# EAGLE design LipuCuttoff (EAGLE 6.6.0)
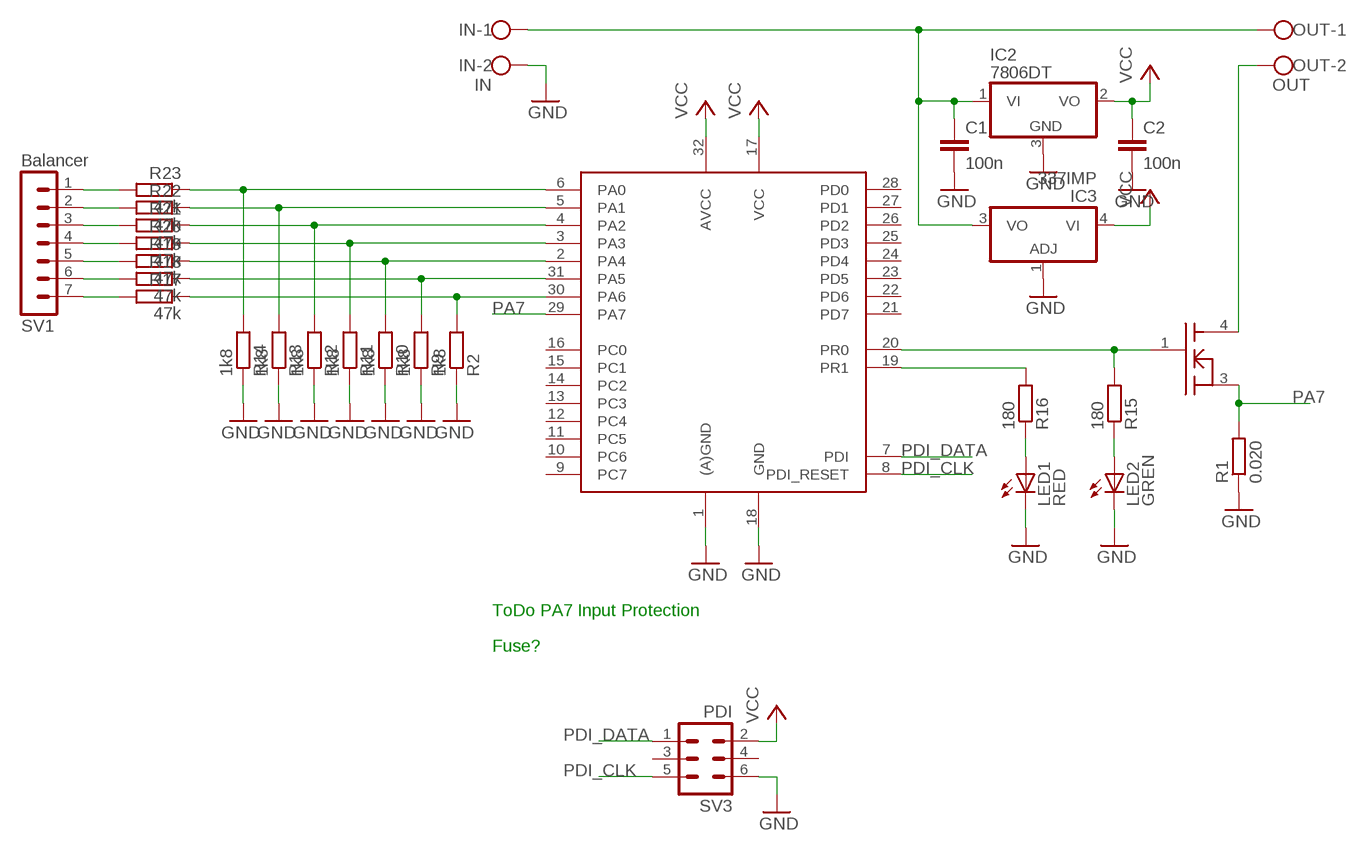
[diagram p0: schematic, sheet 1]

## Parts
C1  100n  C-EUC0805  [C0805]
C2  100n  C-EUC0805  [C0805]
IC2  7806DT  [TO252]
IC3  337IMP  [SOT223]
IN  IN  W237-102  [W237-102]
LED1  RED  LEDSML0805  [SML0805]
LED2  GREN  LEDSML0805  [SML0805]
OUT  OUT  W237-102  [W237-102]
R1  0.020  R-EU_R2512  [R2512]
R2  1k8  R-EU_M0805  [M0805]
R9  1k8  R-EU_M0805  [M0805]
R10  1k8  R-EU_M0805  [M0805]
R11  1k8  R-EU_M0805  [M0805]
R12  1k8  R-EU_M0805  [M0805]
R13  1k8  R-EU_M0805  [M0805]
R14  1k8  R-EU_M0805  [M0805]
R15  180  R-EU_M0805  [M0805]
R16  180  R-EU_M0805  [M0805]
R17  47k  R-EU_M0805  [M0805]
R18  47k  R-EU_M0805  [M0805]
R19  47k  R-EU_M0805  [M0805]
R20  47k  R-EU_M0805  [M0805]
R21  47k  R-EU_M0805  [M0805]
R22  47k  R-EU_M0805  [M0805]
R23  47k  R-EU_M0805  [M0805]
SV1  Balancer  MA07-1  [MA07-1]
SV3  PDI  MA03-2  [MA03-2]
U$1  ATXMEGA8E5  [TQFP-32]
U$2  95N2LH5  [DPAK]

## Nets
GND: C1.2 C2.2 IC2.3(GND) IC3.1(ADJ) IN.2 LED1.C LED2.C R1.1 R2.1 R9.1 R10.1 R11.1 R12.1 R13.1 R14.1 SV3.6 U$1.1((A)GND) U$1.18(GND)
N$1: R17.2 SV1.7
N$2: R18.2 SV1.6
N$3: R9.2 R18.1 U$1.31(PA5)
N$4: R19.2 SV1.5
N$5: R11.2 R20.1 U$1.3(PA3)
N$6: R20.2 SV1.4
N$7: R13.2 R22.1 U$1.5(PA1)
N$8: R21.2 SV1.3
N$9: R22.2 SV1.2
N$10: R23.2 SV1.1
N$12: OUT.2 U$2.4(D)
N$13: C1.1 IC2.1(VI) IC3.3(VO) IN.1 OUT.1
N$15: LED2.A R15.1
N$16: R16.2 U$1.19(PR1)
N$17: LED1.A R16.1
N$18: R15.2 U$1.20(PR0) U$2.1(G)
N$19: R2.2 R17.1 U$1.30(PA6)
N$21: R10.2 R19.1 U$1.2(PA4)
N$23: R12.2 R21.1 U$1.4(PA2)
N$25: R14.2 R23.1 U$1.6(PA0)
PA7: R1.2 U$1.29(PA7) U$2.3(S)
PDI_CLK: SV3.5 U$1.8(PDI_RESET)
PDI_DATA: SV3.1 U$1.7(PDI)
VCC: C2.1 IC2.2(VO) IC3.4(VI) SV3.2 U$1.17(VCC) U$1.32(AVCC)
Unconnected: SV3.3 SV3.4 U$1.9(PC7) U$1.10(PC6) U$1.11(PC5) U$1.12(PC4) U$1.13(PC3) U$1.14(PC2) U$1.15(PC1) U$1.16(PC0) U$1.21(PD7) U$1.22(PD6) U$1.23(PD5) U$1.24(PD4) U$1.25(PD3) U$1.26(PD2) U$1.27(PD1) U$1.28(PD0)

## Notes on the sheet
- ToDo PA7 Input Protection
- Fuse?

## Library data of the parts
C1 C2 = rcl:C-EU: CAPACITOR, European symbol
IC2 = linear:78*: Positive VOLTAGE REGULATOR Source: http://cache.national.com/ds/LM/LM78L05.pdf http://www.fairchildsemi.com/ds/LM/LM7805.pdf
IC3 = linear:*337: Negative VOLTAGE REGULATOR
IN OUT = con-wago-500:W237-102: WAGO SCREW CLAMP; MPN: 237-102; OC_FARNELL: unknown; OC_NEWARK: 70K9898
LED1 LED2 = led:LED: LED
R1 R2 R9-R23 = rcl:R-EU_: RESISTOR, European symbol
SV1 = con-lstb:MA07-1: PIN HEADER; OC_FARNELL: unknown; OC_NEWARK: unknown
SV3 = con-lstb:MA03-2: PIN HEADER; OC_FARNELL: unknown; OC_NEWARK: unknown
U$1 = ATxmega16E5:ATXMEGA8E5
U$2 = Wasle:95N2LH5

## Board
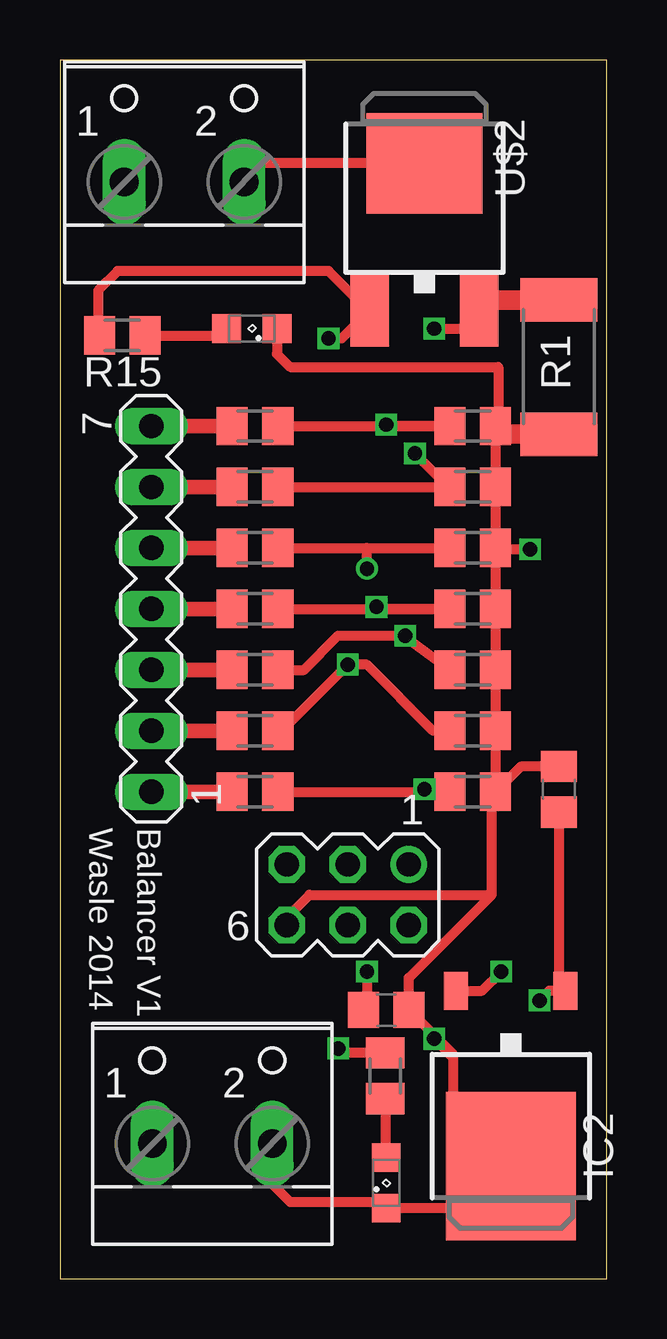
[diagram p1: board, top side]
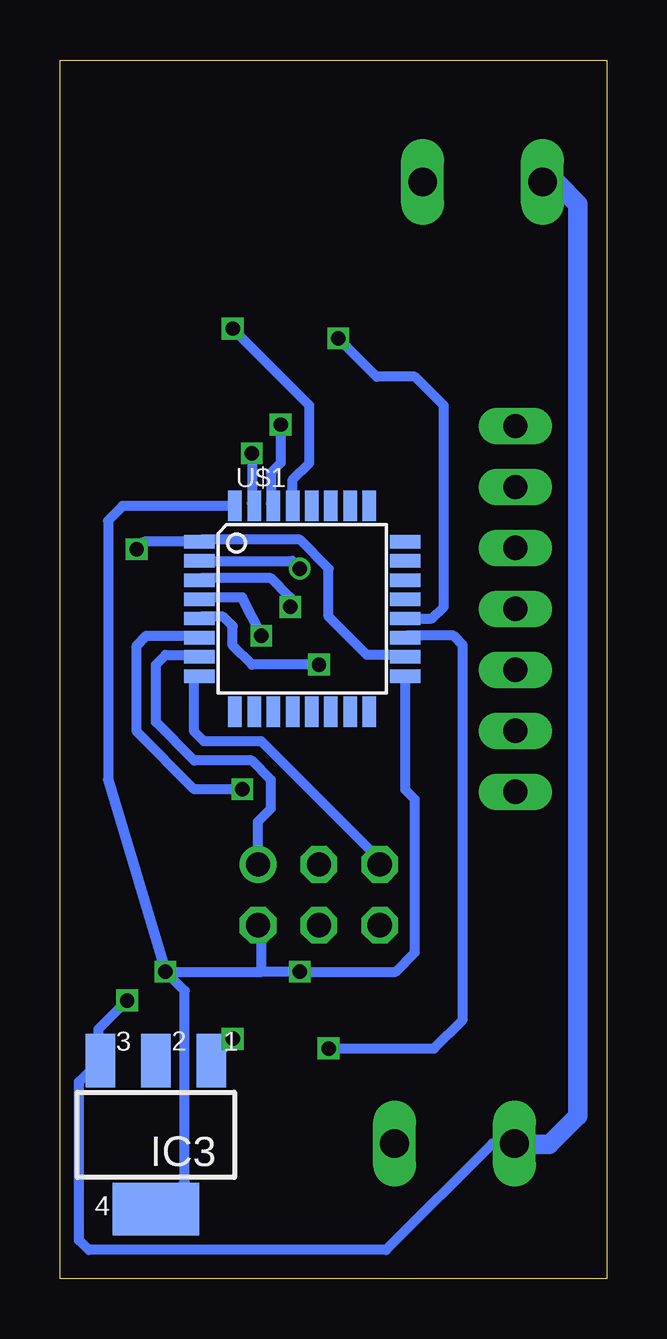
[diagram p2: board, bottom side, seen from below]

Size 22.8 x 50.8 mm. Coordinates in mm from the lower left corner, seen from the top.
Outline: 0,0 22.8,0 22.8,50.8 0,50.8 0,0
Copper layers (1*16): Top 0.035mm / dielectric 1.5mm / Bottom 0.035mm
Design rules "Elecrow_2-layer_eagle_rule": minimum track width 6mil, minimum drill 12mil, track to track 6mil, track to pad 6mil, pad to pad 6mil, via to via 6mil, smd to smd 0mil, copper to edge 10mil, drill to drill 10mil, minimum pad ring 10mil, minimum via ring 6mil, stop-mask expansion 2mil, vias tented up to drill 100mil, thermal gap 10mil

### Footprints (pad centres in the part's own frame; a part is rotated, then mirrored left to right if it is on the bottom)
C0805 = smd 1.3 x 1.5: 1 -0.95,0; 2 0.95,0
TO252 = smd 1 x 1.6: 1 -2.28,-4.8; 2 2.28,-4.8 | smd 5.4 x 6.2: 3 0,2.5
SOT223 = smd 1.219 x 2.235: 1 -2.311,-3.099; 2 0,-3.099; 3 2.311,-3.099 | smd 3.6 x 2.2: 4 0,3.099
W237-102 = drill 1.194 long: 1 -2.5,-1.27; 2 2.5,-1.27
SML0805 = smd 1.2 x 1.2: A 1.05,0; C -1.05,0
R2512 = smd 1.8 x 3.2: 1 -2.8,0; 2 2.8,0
M0805 = smd 1.3 x 1.6: 1 -0.95,0; 2 0.95,0
MA07-1 = drill 1.016 long: 1 -7.62,0; 2 -5.08,0; 3 -2.54,0; 4 0,0; 5 2.54,0; 6 5.08,0; 7 7.62,0
MA03-2 = drill 1.016: 1 -2.54,-1.27 | drill 1.016 octagon: 2 -2.54,1.27; 3 0,-1.27; 4 0,1.27; 5 2.54,-1.27; 6 2.54,1.27
TQFP-32 = smd 1.27 x 0.559: 1 -4.293,2.8; 2 -4.293,2; 3 -4.293,1.2; 4 -4.293,0.4; 5 -4.293,-0.4; 6 -4.293,-1.2; 7 -4.293,-2; 8 -4.293,-2.8; 17 4.293,-2.8; 18 4.293,-2; 19 4.293,-1.2; 20 4.293,-0.4; 21 4.293,0.4; 22 4.293,1.2; 23 4.293,2; 24 4.293,2.8 | smd 0.559 x 1.27: 9 -2.8,-4.293; 10 -2,-4.293; 11 -1.2,-4.293; 12 -0.4,-4.293; 13 0.4,-4.293; 14 1.2,-4.293; 15 2,-4.293; 16 2.8,-4.293; 25 2.8,4.293; 26 2,4.293; 27 1.2,4.293; 28 0.4,4.293; 29 -0.4,4.293; 30 -1.2,4.293; 31 -2,4.293; 32 -2.8,4.293
DPAK = smd 1.6 x 3: 1 -2.28,-4.04; 3 2.28,-4.04 | smd 4.826 x 4.191: 4 0,2.096

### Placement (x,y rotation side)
C1  20.8,20.4 90 top
C2  13.6,11.2 0 top
IC2  18.8,7.2 180 top
IC3  18.8,6 180 bottom
IN  6.35,6.9 0 top
LED1  13.6,4 90 top
LED2  8,39.6 180 top
OUT  5.18,46.99 0 top
R1  20.8,38 90 top
R2  17.21,35.54 180 top
R9  17.21,33 180 top
R10  17.21,30.46 180 top
R11  17.21,27.92 180 top
R12  17.21,25.38 180 top
R13  17.21,22.84 180 top
R14  17.21,20.3 180 top
R15  2.6,39.32 180 top
R16  13.57,8.46 90 top
R17  8.13,35.54 180 top
R18  8.13,33 180 top
R19  8.13,30.46 180 top
R20  8.13,27.92 180 top
R21  8.13,25.38 180 top
R22  8.13,22.84 180 top
R23  8.13,20.3 180 top
SV1  3.81,27.92 90 top
SV3  12,16 180 top
U$1  12.7,27.92 0 bottom
U$2  15.2,44.4 0 top

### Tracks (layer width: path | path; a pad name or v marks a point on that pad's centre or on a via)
GND  (via drill 0.6)
  Top 0.406: R10.1 R9.1 R2.1 18.28,35.66 18.28,38 9.6,38 9.05,38.55 LED2.C | R10.1 R11.1 R12.1 R13.1 R14.1 | IN.2 8.85,3.95 9.6,3.2 13.35,3.2 LED1.C 17.05,2.95 IC2.3 18.8,4.8 16.4,7.2 16.4,9.35 | v19.6,30.4 18.22,30.4 R10.1 | R14.1 18,20.14 18,16 | C1.2 19.21,21.35 R14.1 | 16.4,9.35 C2.2 14.55,12.55 18,16 | 16.4,9.35 16.25,9.35 v15.6,10 | SV3.6 9.46,15.06 10.4,16 18,16
  Top 0.813: R1.1 18.16,35.2 R2.1
  Bottom 0.406: v19.6,30.4 19.28,30.72 U$1.1 16.91,30.8 12.8,30.8 11.6,29.6 11.6,27.6 10,26 8.4,26 8.41,25.99 U$1.18 | v15.6,10 15.6,9.99 IC3.1
N$1
  Top 0.61: SV1.7 R17.2
N$2
  Top 0.61: SV1.6 R18.2
N$3  (via drill 0.6)
  Top 0.406: R18.1 R9.2 16.2,33 v14.8,34.4
  Bottom 0.406: v14.8,34.4 14.8,32.31 U$1.31
N$4
  Top 0.61: SV1.5 R19.2
N$5  (via drill 0.6)
  Top 0.406: R20.1 R11.2 13.28,27.92 v13.2,28
  Bottom 0.406: v13.2,28 13.2,28.4 14,29.2 16.91,29.2 U$1.3
N$6
  Top 0.61: SV1.4 R20.2
N$7  (via drill 0.6)
  Top 0.406: R22.1 9.24,22.84 v12,25.6 12.8,25.6 15.56,22.84 R13.2
  Bottom 0.406: v12,25.6 14.8,25.6 15.6,26.4 15.6,27.2 16,27.6 16.91,27.6 U$1.5
N$8
  Top 0.61: SV1.3 R21.2
N$9
  Top 0.61: SV1.2 R22.2
N$10
  Top 0.61: SV1.1 R23.2
N$12
  Top 0.406: U$2.4 8.46,46.5 OUT.2
N$13  (via drill 0.6)
  Top 0.406: C1.1 20.8,12.28 IC2.1 20.4,12 v20,11.6
  Bottom 0.406: v20,11.6 21.2,10.4 21.2,9.19 IC3.3 22,8.21 22,1.6 21.6,1.2 9.2,1.2 4.77,5.63 IN.1
  Bottom 0.813: OUT.1 2.12,45.72 1.2,44.8 1.2,6.8 2.4,5.6 3.82,5.6 IN.1
N$15
  Top 0.406: R15.1 6.67,39.32 LED2.A
N$16  (via drill 0.6)
  Top 0.406: R16.2 11.79,9.41 v11.6,9.6
  Bottom 0.406: v11.6,9.6 7.2,9.6 6,10.8 6,26.4 6.4,26.8 8.33,26.8 U$1.19
N$17
  Top 0.406: LED1.A 13.6,7.48 R16.1
N$18  (via drill 0.6)
  Top 0.406: R15.2 1.6,39.37 1.6,41.2 2.4,42 11.2,42 12.84,40.36 U$2.1 11.76,39.2 v11.2,39.2
  Bottom 0.406: U$1.20 7.28,27.52 6.8,28 6.8,36.4 8,37.6 9.6,37.6 v11.2,39.2
N$19  (via drill 0.6)
  Top 0.406: R17.1 R2.2 13.66,35.54 v13.6,35.6
  Bottom 0.406: v13.6,35.6 13.6,34 14,33.6 14,32.31 U$1.30
N$21  (via drill 0.6)
  Top 0.406: R19.1 12.8,30.46 | 12.8,30.46 R10.2 | v12.8,29.6 12.8,30.46
  Bottom 0.406: U$1.2 13.12,29.92 v12.8,29.6
N$23  (via drill 0.6)
  Top 0.406: R12.2 14.62,26.58 v14.4,26.8 11.6,26.8 10.18,25.38 R21.1
  Bottom 0.406: v14.4,26.8 15.2,28.4 16.91,28.4 U$1.4
N$25  (via drill 0.6)
  Top 0.406: R23.1 R14.2 15.3,20.3 v15.2,20.4
  Bottom 0.406: v15.2,20.4 17.2,20.4 19.6,22.8 19.6,26.4 19.2,26.8 17.07,26.8 U$1.6
PA7  (via drill 0.6)
  Top 0.406: v15.6,39.6 16.72,39.6 U$2.3
  Top 0.813: R1.2 17.48,40.8 U$2.3
  Bottom 0.406: U$1.29 13.1,33.3 12.4,34 12.4,36.4 v15.6,39.6
PDI_CLK
  Bottom 0.406: SV3.5 9.46,17.46 14.4,22.4 16.8,22.4 17.2,22.8 17.2,24.91 U$1.8
PDI_DATA
  Bottom 0.406: SV3.1 14.54,19.06 14,19.6 14,20.8 14.8,21.6 17.2,21.6 18.8,23.2 18.8,25.6 18.4,26 17.07,26 U$1.7
VCC  (via drill 0.6)
  Top 0.406: v12.8,12.8 12.8,11.35 C2.1 | IC2.2 17.6,12 v18.4,12.8
  Bottom 0.406: U$1.17 8.41,20.39 8,19.98 8,13.6 8.8,12.8 v12.8,12.8 14.4,12.8 | U$1.32 20.19,32.21 20.8,31.6 20.8,20.8 v18.4,12.8 | v18.4,12.8 14.4,12.8 | IC3.4 18.7,2.9 17.6,4 17.6,12 v18.4,12.8 | 14.4,12.8 14.4,14.59 SV3.2

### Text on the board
tNames: Wasle 2014 | Balancer V1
